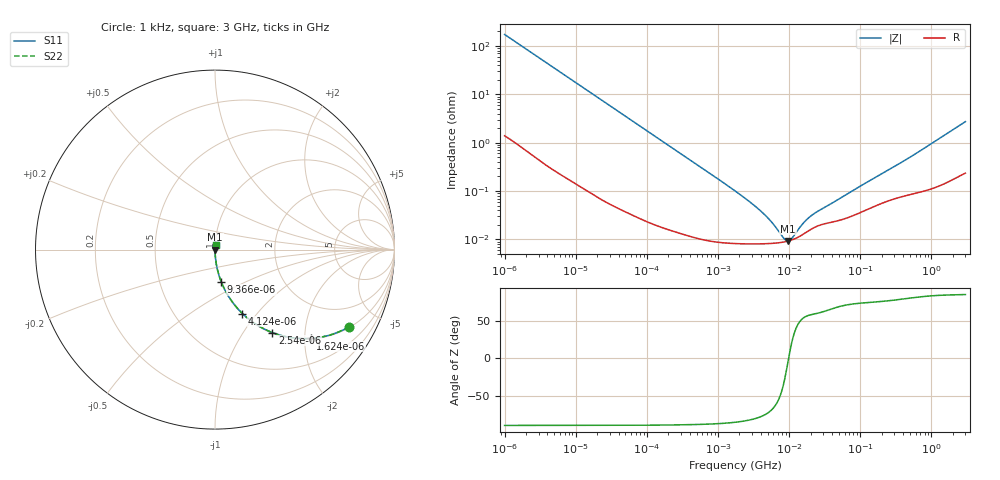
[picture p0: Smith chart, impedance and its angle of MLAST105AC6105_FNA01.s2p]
! MLAST105AC6105_FNA01  S-PARAMETER MODEL  ( Standard Model )
! Model Generated by TAIYO YUDEN Corporation (http://www.ty-top.com)
! Version 1.0
! TAIYO YUDEN Control No. 220601
! Copyright(c) 2015 TAIYO YUDEN CO.,LTD. All Rights Reserved.
! Product Description (link to TY-COMPAS)
! https://ds.yuden.co.jp/TYCOMPAS/or/detail?pn=MLAST105AC6105KFNA01&u=M
! Products Name : Multilayer Ceramic Capacitors
! Characteristics :
!  Capacitance : 1 [uF] , Rated Voltage : 25 [V] , TCC : X6S
!  Case Size : 1.0 x 0.5 / 0.039 x 0.02 [mm/inch] , Thickness : 0.5 / 0.02 [mm/inch]
!  (Conditions: Temperature = 25 [degC] , DC Bias Voltage = 0 [V])
! External Node Assignments :
!  1  o---| |---o  2
! GND o---------o GND
! Frequency Range : 1kHz  -  3GHz  [ 401 STEP ]
# MHZ S RI R 50
! Freq[MHz].  S11 Real  S11 Imag  S21 Real  S21 Imag  S12 Real  S12 Imag  S22 Real  S22 Imag
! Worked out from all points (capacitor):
!   401 points, 1 kHz to 3 GHz, reference 50 ohm
!   read as one part in series: C = 919 nF near 1.077 kHz
!   lowest |Z| = 9.25 mohm at 9.626 MHz (marker M1)
!   series resonance near 9.824 MHz, so ESL is about 290 pH
!   S11 on the Smith chart (normalised r, x): 1 kHz: 1.03, -3.46; 1.624 kHz: 1.02, -2.14; 2.54 kHz: 1.01, -1.37; 4.124 kHz: 1.01, -0.84; 9.366 kHz: 1.00, -0.37; 3 GHz: 1.00, +0.05
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0.001  0.7475 -0.4305  0.2525 0.4305  0.2525 0.4305  0.7475 -0.4305
0.001624  0.5324 -0.495  0.4676 0.495  0.4676 0.495  0.5324 -0.495
0.00254  0.3201 -0.4627  0.6799 0.4627  0.6799 0.4627  0.3201 -0.4627
0.004124  0.1532 -0.3564  0.8468 0.3564  0.8468 0.3564  0.1532 -0.3564
0.005988  0.0799 -0.2674  0.9201 0.2674  0.9201 0.2674  0.0799 -0.2674
0.009366  0.035 -0.1798  0.965 0.1798  0.965 0.1798  0.035 -0.1798
0.01216  0.0214 -0.1407  0.9786 0.1407  0.9786 0.1407  0.0214 -0.1407
0.033275  0.00327 -0.0526  0.9967 0.0526  0.9967 0.0526  0.00327 -0.0526
0.147855  0.000329 -0.012  0.9997 0.012  0.9997 0.012  0.000329 -0.012
1.732051  8.3e-05 -0.001  0.9999 0.001  0.9999 0.001  8.3e-05 -0.001
2.812335  8.1e-05 -0.000587  0.9999 0.000587  0.9999 0.000587  8.1e-05 -0.000587
4.083148  8.11e-05 -0.000365  0.9999 0.000365  0.9999 0.000365  8.11e-05 -0.000365
5.711239  8.27e-05 -0.000209  0.9999 0.000209  0.9999 0.000209  8.27e-05 -0.000209
8.291982  8.79e-05 -6.27e-05  0.9999 6.27e-05  0.9999 6.27e-05  8.79e-05 -6.27e-05
9.625639  9.22e-05 -7.45e-06  0.9999 7.45e-06  0.9999 7.45e-06  9.22e-05 -7.45e-06
10.37087  9.51e-05 2e-05  0.9999 -2e-05  0.9999 -2e-05  9.51e-05 2e-05
11.1738  9.87e-05 4.75e-05  0.9999 -4.75e-05  0.9999 -4.75e-05  9.87e-05 4.75e-05
15.62917  0.000127 0.000171  0.9999 -0.000171  0.9999 -0.000171  0.000127 0.000171
21.06097  0.000167 0.000273  0.9998 -0.000273  0.9998 -0.000273  0.000167 0.000273
256.0921  0.000643 0.00272  0.9994 -0.00272  0.9994 -0.00272  0.000643 0.00272
560.3316  0.000907 0.00548  0.9991 -0.00548  0.9991 -0.00548  0.000907 0.00548
3000  0.00307 0.027  0.9969 -0.027  0.9969 -0.027  0.00307 0.027
